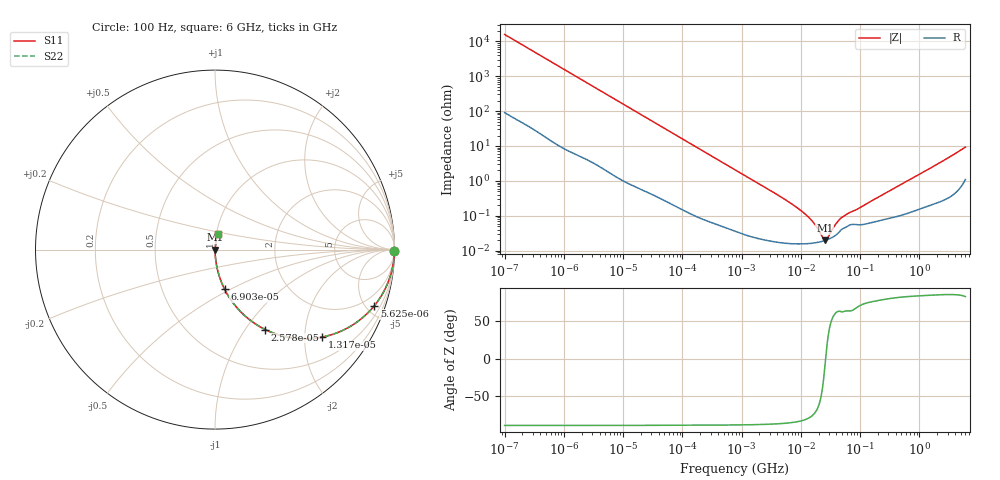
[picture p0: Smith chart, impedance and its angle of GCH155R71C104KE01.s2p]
!Murata Part Number: GCH155R71C104KE01
!These Parameters are Measured in Series Mode Connection
!Data Generated on Jun 19, 2026
!  o--ll--o
!Port1  Port2
!  o------o
!Operation Temp=25[degC], DC Bias Voltage=0[V]
!Freq. Start=100[Hz] Stop=6[GHz] 401[Steps]
# Hz S RI R 50
!Freq.(Hz) S11(Real) S11(Imag) S21(Real) S21(Imag) S12(Real) S12(Imag) S22(Real) S22(Imag)
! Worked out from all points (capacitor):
!   401 points, 100 Hz to 6 GHz, reference 50 ohm
!   read as one part in series: C = 101 nF near 109 Hz
!   lowest |Z| = 19.9 mohm at 25.46 MHz (marker M1)
!   series resonance near 26.24 MHz, so ESL is about 360 pH
!   S11 on the Smith chart (normalised r, x): 100 Hz: open; 5.625 kHz: 1.04, -5.66; 13.17 kHz: 1.02, -2.43; 25.78 kHz: 1.01, -1.24; 69.03 kHz: 1.00, -0.47; 6 GHz: 1.02, +0.18
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100  0.9999 -0.00637  7.75e-05 0.00637  7.75e-05 0.00637  0.9999 -0.00637
627  0.9982 -0.0396  0.00178 0.0396  0.00178 0.0396  0.9982 -0.0396
2008  0.9835 -0.1245  0.0165 0.1245  0.0165 0.1245  0.9835 -0.1245
5625  0.8876 -0.3127  0.1124 0.3127  0.1124 0.3127  0.8876 -0.3127
8416  0.7808 -0.4106  0.2192 0.4106  0.2192 0.4106  0.7808 -0.4106
13169  0.5948 -0.4877  0.4052 0.4877  0.4052 0.4877  0.5948 -0.4877
25777  0.2801 -0.4453  0.7199 0.4453  0.7199 0.4453  0.2801 -0.4453
40335  0.1388 -0.3417  0.8612 0.3417  0.8612 0.3417  0.1388 -0.3417
69028  0.0534 -0.2204  0.9466 0.2204  0.9466 0.2204  0.0534 -0.2204
193316  0.00782 -0.083  0.9922 0.083  0.9922 0.083  0.00782 -0.083
774597  0.000803 -0.0211  0.9992 0.0211  0.9992 0.0211  0.000803 -0.0211
6644369  0.000165 -0.00233  0.9998 0.00233  0.9998 0.00233  0.000165 -0.00233
1.087309e7  0.000159 -0.00126  0.9998 0.00126  0.9998 0.00126  0.000159 -0.00126
1.555665e7  0.000164 -0.00069  0.9998 0.00069  0.9998 0.00069  0.000164 -0.00069
2.327686e7  0.000187 -0.000151  0.9998 0.000151  0.9998 0.000151  0.000187 -0.000151
2.545746e7  0.000196 -3.8e-05  0.9998 3.8e-05  0.9998 3.8e-05  0.000196 -3.8e-05
2.784235e7  0.000206 7.5e-05  0.9998 -7.5e-05  0.9998 -7.5e-05  0.000206 7.5e-05
3.80911e7  0.000271 0.00048  0.9997 -0.00048  0.9997 -0.00048  0.000271 0.00048
4.983056e7  0.000418 0.000807  0.9996 -0.000807  0.9996 -0.000807  0.000418 0.000807
3.124326e8  0.000869 0.00504  0.9991 -0.00504  0.9991 -0.00504  0.000869 0.00504
1.95892e9  0.00316 0.0291  0.9968 -0.0291  0.9968 -0.0291  0.00316 0.0291
6e9  0.0189 0.0895  0.9811 -0.0895  0.9811 -0.0895  0.0189 0.0895
